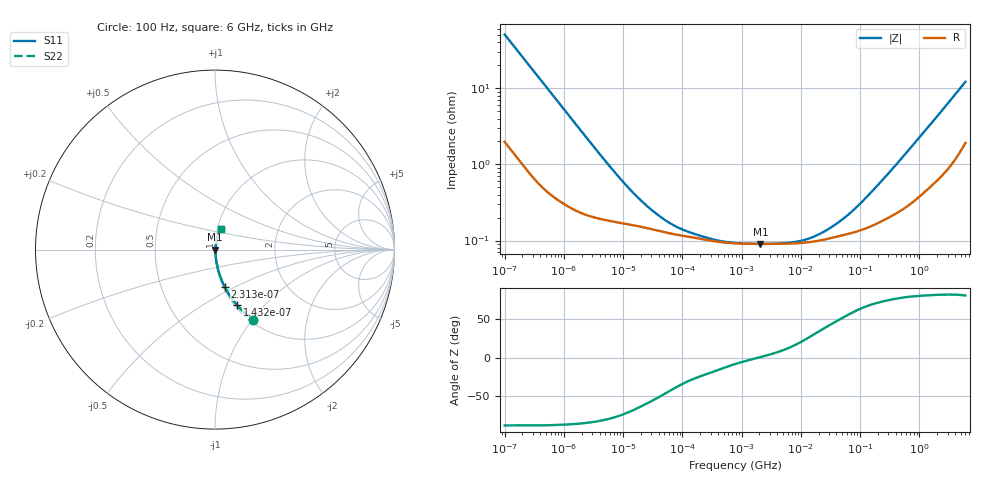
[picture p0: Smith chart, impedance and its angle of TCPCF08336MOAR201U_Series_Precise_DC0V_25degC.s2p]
! TCPCF08336MOAR201U Polymer Tantalum Capacitor Sparameter Model
! Model Generated by Samsung Electro-Mechanics
! Samsung Sparameter Version 5.0
! Date : Oct-10-2024
! Products : Polymer Tantalum Capacitor
! Characteristics :
!  Nominal Capacitance = 33uF
!  Capacitance Tolerance = +/-20%
!  ESR = 200 mohm max at 100kHz
!  Rated Voltage = 8Vdc
!  Size = 0805(unit:inch), 2012(unit:mm)
!  Length = 2.00+/-0.20mm
!  Width = 1.25+/-0.20mm
!  Thickness = 0.70+/-0.10mm
!  Lineup = Conductive Polymer Type
!  Feature = PCF
!  Measurement Temperature : 25degC.
!  DC bias Value = 0V
!  Frequency : 100Hz ~ 6GHz
! External Node Assignments :
!  1  o---||---o  2
# MHz S RI R 50.0
! Freq.  Real(S11)  Im(S11)  Real(S12)  Im(S12)  Real(S21)  Im(S21)  Real(S22)  Im(S22)
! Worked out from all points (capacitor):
!   300 points, 100 Hz to 6 GHz, reference 50 ohm
!   read as one part in series: C = 31.2 uF near 106.2 Hz
!   lowest |Z| = 90.4 mohm at 2.081 MHz (marker M1)
!   series resonance near 1.863 MHz, so ESL is about 230 pH
!   S11 on the Smith chart (normalised r, x): 100 Hz: 1.04, -1.01; 143.2 Hz: 1.03, -0.71; 231.3 Hz: 1.02, -0.45; 6 GHz: 1.04, +0.24
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0.0001  0.2137 -0.3909  0.7863 0.3909  0.7863 0.3909  0.2137 -0.3909
0.0001432463  0.1225 -0.309  0.8775 0.309  0.8775 0.309  0.1225 -0.309
0.00023131  0.055 -0.2094  0.945 0.2094  0.945 0.2094  0.055 -0.2094
0.0006031378  0.0114 -0.0858  0.9886 0.0858  0.9886 0.0858  0.0114 -0.0858
0.001998454  0.003 -0.0267  0.997 0.0267  0.997 0.0267  0.003 -0.0267
0.005874137  0.0019 -0.00935  0.9981 0.00935  0.9981 0.00935  0.0019 -0.00935
0.01205343  0.00166 -0.00473  0.9983 0.00473  0.9983 0.00473  0.00166 -0.00473
0.02194065  0.0015 -0.00276  0.9985 0.00276  0.9985 0.00276  0.0015 -0.00276
0.03993819  0.00134 -0.00165  0.9987 0.00165  0.9987 0.00165  0.00134 -0.00165
0.0726988  0.00121 -0.001  0.9988 0.001  0.9988 0.001  0.00121 -0.001
0.1323324  0.00112 -0.000633  0.9989 0.000633  0.9989 0.000633  0.00112 -0.000633
0.3450549  0.000979 -0.000309  0.999 0.000309  0.999 0.000309  0.000979 -0.000309
0.7981464  0.000918 -0.000126  0.9991 0.000126  0.9991 0.000126  0.000918 -0.000126
2.081156  0.000903 1.51e-05  0.9991 -1.51e-05  0.9991 -1.51e-05  0.000903 1.51e-05
6.895764  0.000914 0.000232  0.9991 -0.000232  0.9991 -0.000232  0.000914 0.000232
15.95059  0.000966 0.000547  0.999 -0.000547  0.999 -0.000547  0.000966 0.000547
30.82687  0.00107 0.000981  0.9989 -0.000981  0.9989 -0.000981  0.00107 0.000981
63.25518  0.00123 0.00181  0.9988 -0.00181  0.9988 -0.00181  0.00123 0.00181
122.25  0.00144 0.00325  0.9986 -0.00325  0.9986 -0.00325  0.00144 0.00325
318.7652  0.0021 0.00771  0.9979 -0.00771  0.9979 -0.00771  0.0021 0.00771
1922.593  0.00755 0.0402  0.9925 -0.0402  0.9925 -0.0402  0.00755 0.0402
6000  0.0321 0.1137  0.9679 -0.1137  0.9679 -0.1137  0.0321 0.1137
